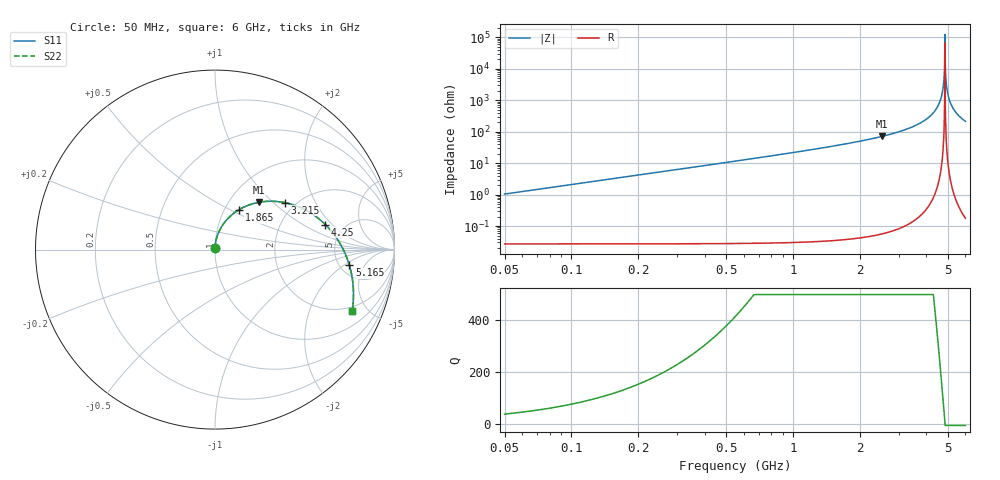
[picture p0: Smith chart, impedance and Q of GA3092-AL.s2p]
! Coilcraft GA3092-AL Air Core Inductor
! 01 July 2008
# MHZ S MA R 50
!Freq  MagS11  AngS11  MagS21  AngS21  MagS12  AngS12  MagS22  AngS22
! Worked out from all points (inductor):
!   398 points, 50 MHz to 6 GHz, reference 50 ohm
!   read as 1/Y11, port 2 shorted: L = 3.31 nH near 65 MHz
!   highest Q = 1.26e+03 at 2.525 GHz (marker M1), where L = 4.47 nH
!   self-resonance near 4.85 GHz
!   S11 on the Smith chart (normalised r, x): 50 MHz: 1.00, +0.01; 1.865 GHz: 1.17, +0.56; 3.215 GHz: 1.77, +1.18; 4.25 GHz: 3.59, +1.66; 5.165 GHz: 6.10, -2.48; 6 GHz: 1.72, -3.96
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50  0.006712 86.9  0.9997 -0.8  0.9997 -0.8  0.006716 86.9
65  0.008723 87.2  0.9997 -1.0  0.9997 -1.0  0.008729 87.2
95  0.01275 87.3  0.9996 -1.5  0.9996 -1.5  0.01275 87.3
155  0.0208 86.8  0.9995 -2.5  0.9995 -2.5  0.02081 86.8
230  0.03087 85.8  0.9993 -3.7  0.9993 -3.7  0.03089 85.8
335  0.04499 84.2  0.9987 -5.4  0.9987 -5.4  0.04502 84.2
470  0.0632 82.2  0.9977 -7.6  0.9977 -7.6  0.06324 82.2
620  0.08353 79.8  0.9962 -10.0  0.9962 -10.0  0.08358 79.8
815  0.1101 76.6  0.9936 -13.2  0.9936 -13.2  0.1102 76.6
1055  0.1433 72.7  0.9894 -17.2  0.9894 -17.2  0.1434 72.7
1415  0.194 66.7  0.9807 -23.2  0.9807 -23.2  0.1941 66.7
1865  0.2593 59.0  0.9655 -31.0  0.9655 -31.0  0.2595 59.0
2045  0.2861 55.8  0.9579 -34.1  0.9579 -34.1  0.2863 55.8
2525  0.3595 47.1  0.9328 -42.8  0.9328 -42.8  0.3597 47.1
3035  0.4399 37.4  0.8977 -52.5  0.8977 -52.5  0.4402 37.4
3215  0.4687 33.9  0.883 -56.0  0.883 -56.0  0.4689 33.9
4025  0.5965 17.5  0.8022 -72.5  0.8022 -72.5  0.5968 17.5
4250  0.6305 12.8  0.7758 -77.2  0.7758 -77.2  0.6308 12.8
5015  0.7358 -3.5  0.6767 -93.5  0.6767 -93.5  0.7361 -3.5
5165  0.754 -6.7  0.6564 -96.7  0.6564 -96.7  0.7543 -6.7
5585  0.8 -15.6  0.5995 -105.6  0.5995 -105.6  0.8003 -15.6
6000  0.8378 -24.2  0.5454 -114.2  0.5454 -114.2  0.8381 -24.2
